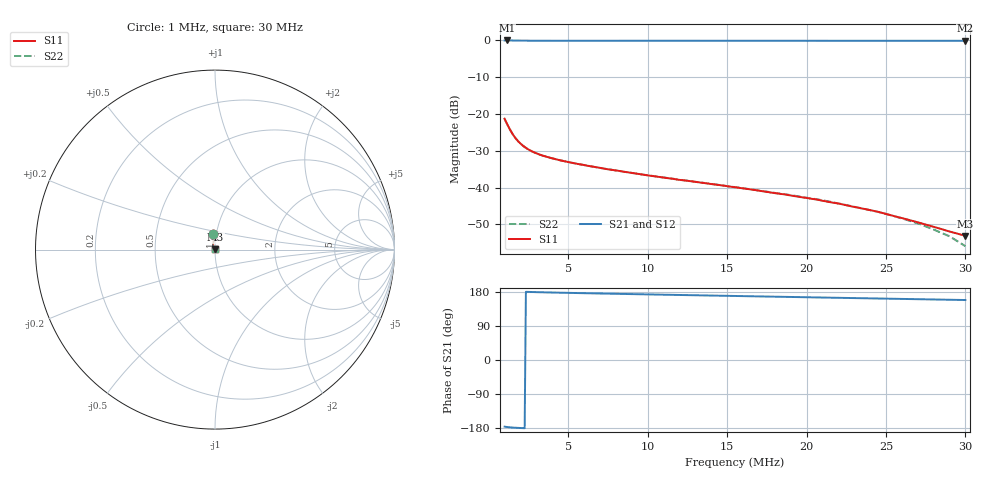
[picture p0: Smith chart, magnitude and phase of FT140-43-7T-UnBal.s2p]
! ListType=Log
!!FT140-43 7T Balun Unbalanced
# MHZ S RI R 50
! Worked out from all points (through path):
!   101 points, 1 MHz to 30 MHz, reference 50 ohm
!   highest |S21| = -0.07 dB at 1.146 MHz (marker M1); lowest = -0.2 dB at 30 MHz (marker M2)
!   lowest |S11| = -53.1 dB at 30 MHz (marker M3), VSWR 1.00, Z = 50.2 + j0.106 ohm
!   |S11| at or under -10 dB: start of sweep to end of sweep
!   |S22| runs from -55.9 to -21.3 dB; largest |S21 - S12| = 0.00017
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1  -0.00863 0.0855  -0.9886 -0.0698  -0.9887 -0.0697  -0.00867 0.0854
1.145737  -0.00703 0.0733  -0.9899 -0.0556  -0.99 -0.0555  -0.00709 0.0732
1.453729  -0.00658 0.0551  -0.9898 -0.0332  -0.9899 -0.0331  -0.00667 0.0551
1.723215  -0.00769 0.0451  -0.9882 -0.0195  -0.9883 -0.0195  -0.00777 0.0451
1.908328  -0.00855 0.0404  -0.9871 -0.0123  -0.9872 -0.0122  -0.00863 0.0403
2.113327  -0.00927 0.0364  -0.986 -0.00555  -0.986 -0.00553  -0.00936 0.0364
2.505087  -0.0103 0.0311  -0.9844 0.00492  -0.9844 0.00494  -0.0104 0.0311
3.178493  -0.0109 0.0259  -0.9825 0.019  -0.9827 0.019  -0.011 0.0259
3.767708  -0.0109 0.0233  -0.9816 0.0293  -0.9817 0.0294  -0.0109 0.0232
4.780527  -0.0101 0.0204  -0.9806 0.0453  -0.9807 0.0453  -0.0101 0.0203
5.862773  -0.00901 0.0184  -0.9798 0.0611  -0.9799 0.0611  -0.0091 0.0183
7.438777  -0.00734 0.0162  -0.9784 0.0831  -0.9785 0.0831  -0.00747 0.0162
10.81396  -0.00457 0.0131  -0.9737 0.1281  -0.9738 0.1281  -0.00479 0.013
15.72057  -0.00176 0.00978  -0.9631 0.1908  -0.9632 0.1909  -0.00214 0.00975
20.63659  0.000104 0.00686  -0.9484 0.2516  -0.9485 0.2517  -0.000476 0.00692
22.08922  0.000531 0.006  -0.9433 0.2693  -0.9435 0.2693  -0.000117 0.00603
24.46211  0.00111 0.00458  -0.9344 0.2978  -0.9345 0.2979  0.000357 0.00468
25.30843  0.00128 0.00401  -0.931 0.3079  -0.9311 0.3079  0.000479 0.00417
27.08991  0.00163 0.00291  -0.9235 0.329  -0.9237 0.329  0.000711 0.00314
28.02714  0.00176 0.00233  -0.9194 0.34  -0.9195 0.34  0.000762 0.00256
28.9968  0.00185 0.00173  -0.915 0.3513  -0.9151 0.3513  0.000836 0.00201
30  0.00194 0.00105  -0.9103 0.363  -0.9104 0.363  0.000862 0.00135
